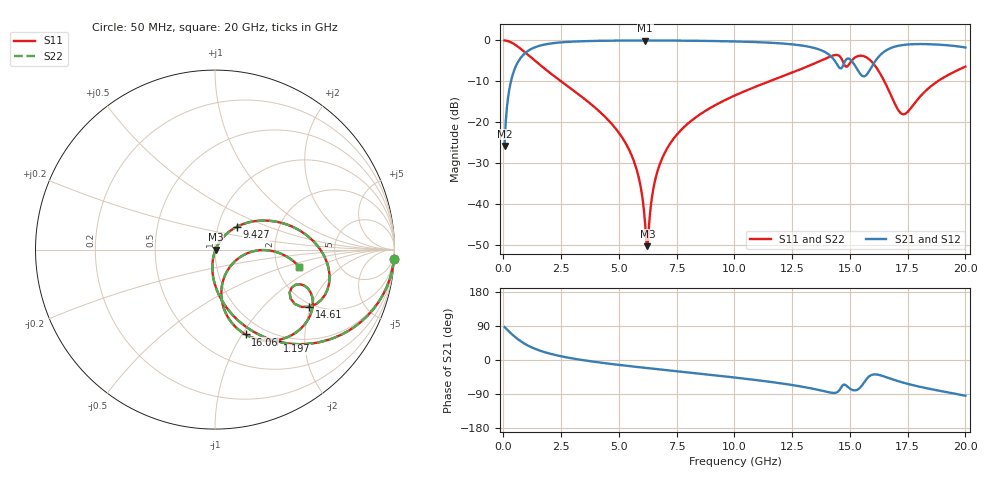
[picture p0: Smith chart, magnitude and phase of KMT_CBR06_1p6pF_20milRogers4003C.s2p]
! Data measured by Modelithics Inc. support@modelithics.com 813-866-6335
! KEMET CBR0603 1.6pF, Pad Width= 0.851mm, Pad Length= 0.64mm, Pad Gap= 0.62mm, 20mil Rogers 4003C substrate Data, January 2022
# hz S ma R 50
! 2 Port Network Data from SP1.SP block
! freq  magS11  angS11  magS21  angS21  magS12  angS12  magS22  angS22
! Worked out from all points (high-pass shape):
!   401 points, 50 MHz to 20 GHz, reference 50 ohm
!   highest |S21| = -0.03 dB at 6.135 GHz (marker M1); lowest = -25.8 dB at 50 MHz (marker M2)
!   |S21| within 3 dB of the highest: 953.6 MHz to 13.98 GHz (13.02 GHz wide, 174 % of centre); 16.42 GHz to end of sweep
!   lowest |S11| = -50.3 dB at 6.234 GHz (marker M3), VSWR 1.01, Z = 50.3 - j0.035 ohm
!   |S11| at or under -10 dB: 2.497 GHz to 11.51 GHz (9.013 GHz wide, 129 % of centre); 16.49 GHz to 18.8 GHz (2.305 GHz wide, 13.1 % of centre)
!   |S22| runs from -50.3 to 0.0 dB; largest |S21 - S12| = 0
!   S11 on the Smith chart (normalised r, x): 50 MHz: 1, -37; 1.197 GHz: 0.90, -1.49; 9.427 GHz: 1.23, +0.32; 14.61 GHz: 1.90, -1.94; 16.06 GHz: 0.82, -1.04; 20 GHz: 2.65, -0.65
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5e7  0.9987 -3.1  0.05119 86.9  0.05119 86.9  0.9987 -3.1
2.495e8  0.9686 -15.2  0.2481 74.7  0.2481 74.7  0.9686 -15.2
4.49e8  0.9073 -26.4  0.4195 63.6  0.4195 63.6  0.9073 -26.4
1.197125e9  0.6183 -55.8  0.7844 34.1  0.7844 34.1  0.6183 -55.8
3.391625e9  0.2045 -89.2  0.9765 0.1  0.9765 0.1  0.2045 -89.2
5.4365e9  0.04634 -102.6  0.996 -16.0  0.996 -16.0  0.04634 -102.6
5.885375e9  0.01951 -100.6  0.9967 -19.1  0.9967 -19.1  0.01951 -100.6
6.13475e9  0.005698 -79.8  0.9968 -20.7  0.9968 -20.7  0.005698 -79.8
6.2345e9  0.003064 -6.5  0.9968 -21.4  0.9968 -21.4  0.003064 -6.5
6.73325e9  0.02872 59.1  0.9962 -24.7  0.9962 -24.7  0.02872 59.1
7.680875e9  0.07989 56.7  0.993 -30.8  0.993 -30.8  0.07989 56.7
9.4265e9  0.1767 46.2  0.9791 -42.2  0.9791 -42.2  0.1767 46.2
1.0025e10  0.2128 42.2  0.9711 -46.3  0.9711 -46.3  0.2128 42.2
1.336662e10  0.5084 9.9  0.8202 -75.4  0.8202 -75.4  0.5084 9.9
1.426438e10  0.6525 -12.3  0.6032 -86.8  0.6032 -86.8  0.6525 -12.3
1.46135e10  0.6136 -31.3  0.4545 -73.1  0.4545 -73.1  0.6136 -31.3
1.496262e10  0.5119 -22.1  0.5976 -73.7  0.5976 -73.7  0.5119 -22.1
1.536162e10  0.645 -34.8  0.4232 -77.1  0.4232 -77.1  0.645 -34.8
1.605988e10  0.5024 -70.2  0.5377 -38.0  0.5377 -38.0  0.5024 -70.2
1.670825e10  0.2362 -81.4  0.7935 -48.2  0.7935 -48.2  0.2362 -81.4
1.735662e10  0.1256 -36.9  0.8831 -60.6  0.8831 -60.6  0.1256 -36.9
2e10  0.479 -11.4  0.8193 -94.3  0.8193 -94.3  0.479 -11.4
